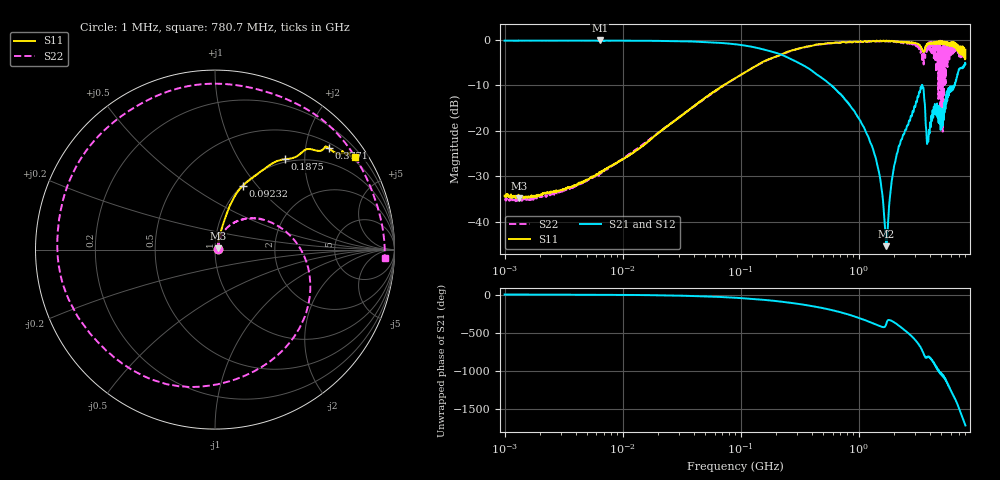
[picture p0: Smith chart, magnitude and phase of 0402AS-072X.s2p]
!s-Parameter Generated by FASTRON Sdn. Bhd.
!FASTRON P/N : 0402AS-072X
!Keysight Technologies: E5071C_MY46733604_B.14.02
!Date: Mon Dec 01 10:48:24 2025
!Version  :Rev00  Mon Dec 01 10:48:24 2025
!Data & Calibration Information:
!Freq  S11:SOLT2(ON)  S21:SOLT2(ON)  S12:SOLT2(ON)  S22:SOLT2(ON)
!PortZ  Port1:50+j0  Port2:50+j0
!When reading reference impedance value at option line is always used.
! Remarks : This data is being provided solely for informational purposes.
# Hz S dB R 50
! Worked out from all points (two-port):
!   1601 points, 1 MHz to 8 GHz, reference 50 ohm
!   highest |S21| = -0.12 dB at 6.4 MHz (marker M1); lowest = -45.4 dB at 1.71 GHz (marker M2)
!   |S21| within 3 dB of the highest: start of sweep to 214.5 MHz
!   lowest |S11| = -34.9 dB at 1.323 MHz (marker M3), VSWR 1.04, Z = 51.7 + j0.652 ohm
!   |S11| at or under -10 dB: start of sweep to 71.39 MHz
!   |S22| runs from -35.5 to -0.2 dB; largest |S21 - S12| = 0.011
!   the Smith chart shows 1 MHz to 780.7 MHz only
!   S11 on the Smith chart (normalised r, x): 1 MHz: 1.04, +0.01; 92.32 MHz: 1.01, +0.84; 187.5 MHz: 0.95, +1.61; 377.1 MHz: 0.61, +2.50; 780.7 MHz: 0.39, +3.28
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1000000  -34.30 16.8  -0.17 -0.5  -0.15 -0.5  -35.10 16.9
1323440  -34.90 20.5  -0.17 -0.7  -0.14 -0.7  -35.20 18.2
4479405  -31.30 50.3  -0.16 -2.3  -0.14 -2.2  -31.60 50.1
6400096  -29.10 58.4  -0.12 -3.1  -0.17 -3.0  -29.20 54.4
2.00676e7  -20.50 71.9  -0.22 -10.0  -0.20 -9.9  -20.40 65.4
8.994653e7  -8.42 67.0  -0.96 -42.4  -0.95 -42.4  -8.44 19.9
9.232141e7  -8.24 66.5  -0.99 -43.5  -0.98 -43.4  -8.26 18.3
1.875349e8  -3.92 52.2  -2.65 -81.5  -2.64 -81.5  -3.94 -40.5
3.771449e8  -1.41 41.6  -6.30 -145.0  -6.29 -145.0  -1.40 -154.0
4.006501e8  -1.31 38.8  -6.78 -152.0  -6.76 -152.0  -1.23 -166.0
5.934802e8  -0.75 34.4  -10.10 155.0  -10.10 155.0  -0.68 93.6
7.806701e8  -0.57 33.5  -13.40 107.0  -13.40 107.0  -0.48 -2.9
1.114569e9  -0.28 38.1  -19.40 27.4  -19.40 27.2  -0.46 -170.0
1.334081e9  -0.22 44.7  -24.50 -20.6  -24.50 -20.8  -0.37 83.4
1.709681e9  -0.15 56.4  -45.40 -24.2  -45.30 -23.9  -0.35 -96.5
1.7949e9  -0.20 58.2  -37.50 25.8  -37.50 26.0  -0.38 -137.0
2.061212e9  -0.42 64.4  -26.00 -18.4  -26.00 -18.3  -0.39 94.6
2.428208e9  -0.55 70.9  -20.60 -103.0  -20.60 -103.0  -0.42 -86.9
2.809687e9  -0.60 81.4  -16.80 171.0  -16.80 171.0  -0.54 88.8
3.162936e9  -0.88 90.1  -12.40 80.3  -12.40 80.0  -1.66 -93.5
3.548043e9  -2.38 109.0  -11.20 -61.7  -11.10 -62.0  -5.40 78.2
8e9  -2.18 -115.0  -5.27 83.8  -5.30 83.5  -4.22 122.0
